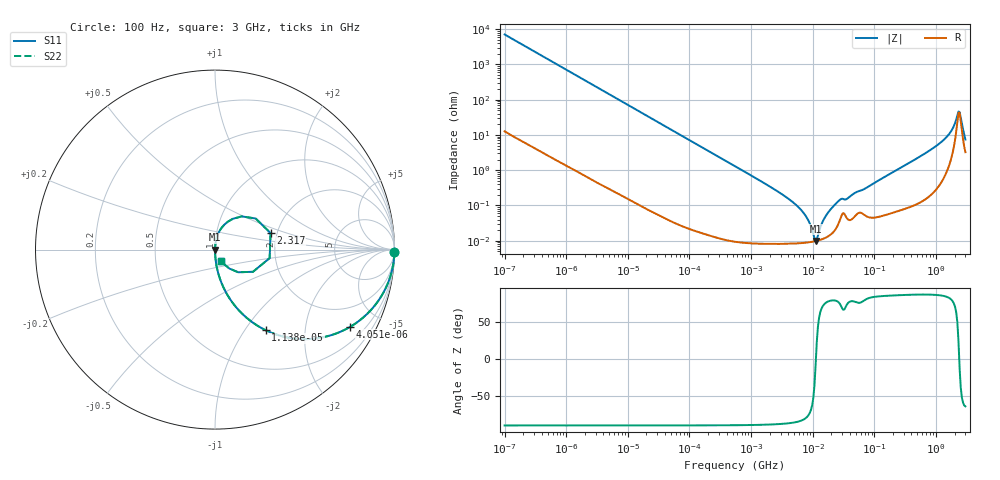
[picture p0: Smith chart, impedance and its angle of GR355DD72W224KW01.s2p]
!Murata Part Number: GR355DD72W224KW01
!These Parameters are Measured in Series Mode Connection
!Data Generated on Mar 13, 2026
!  o--ll--o
!Port1  Port2
!  o------o
!Operation Temp=25[degC], DC Bias Voltage=0[V]
!Freq. Start=100[Hz] Stop=3[GHz] 401[Steps]
# Hz S RI R 50
!Freq.(Hz) S11(Real) S11(Imag) S21(Real) S21(Imag) S12(Real) S12(Imag) S22(Real) S22(Imag)
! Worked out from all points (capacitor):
!   401 points, 100 Hz to 3 GHz, reference 50 ohm
!   read as one part in series: C = 225 nF near 109 Hz
!   lowest |Z| = 9.85 mohm at 11.14 MHz (marker M1)
!   series resonance near 11.26 MHz, so ESL is about 890 pH
!   S11 on the Smith chart (normalised r, x): 100 Hz: open; 4.051 kHz: 1.01, -3.51; 11.38 kHz: 1.00, -1.25; 2.317 GHz: 1.85, +0.38; 3 GHz: 1.06, -0.13
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100  0.9998 -0.0141  0.000225 0.0141  0.000225 0.0141  0.9998 -0.0141
536  0.9942 -0.0751  0.00581 0.0751  0.00581 0.0751  0.9942 -0.0751
1788  0.94 -0.2365  0.06 0.2365  0.06 0.2365  0.94 -0.2365
4051  0.7546 -0.4293  0.2454 0.4293  0.2454 0.4293  0.7546 -0.4293
11382  0.2818 -0.4488  0.7182 0.4488  0.7182 0.4488  0.2818 -0.4488
31977  0.0478 -0.2122  0.9522 0.2122  0.9522 0.2122  0.0478 -0.2122
102221  0.00507 -0.0695  0.9949 0.0695  0.9949 0.0695  0.00507 -0.0695
547723  0.000263 -0.013  0.9997 0.013  0.9997 0.013  0.000263 -0.013
4919190  8.45e-05 -0.00118  0.9999 0.00118  0.9999 0.00118  8.45e-05 -0.00118
7565221  8.79e-05 -0.000521  0.9999 0.000521  0.9999 0.000521  8.79e-05 -0.000521
9794414  9.34e-05 -0.000179  0.9999 0.000179  0.9999 0.000179  9.34e-05 -0.000179
1.11444e7  9.76e-05 -1.29e-05  0.9999 1.29e-05  0.9999 1.29e-05  9.76e-05 -1.29e-05
1.214626e7  0.000101 9.78e-05  0.9999 -9.78e-05  0.9999 -9.78e-05  0.000101 9.78e-05
1.641694e7  0.000123 0.000502  0.9999 -0.000502  0.9999 -0.000502  0.000123 0.000502
2.635803e7  0.000315 0.00131  0.9997 -0.00131  0.9997 -0.00131  0.000315 0.00131
1.751444e8  0.000637 0.00767  0.9994 -0.00767  0.9994 -0.00767  0.000637 0.00767
1.163803e9  0.00739 0.0583  0.9926 -0.0583  0.9926 -0.0583  0.00739 0.0583
1.789813e9  0.0388 0.124  0.9612 -0.124  0.9612 -0.124  0.0388 0.124
2.126076e9  0.1486 0.185  0.8514 -0.185  0.8514 -0.185  0.1486 0.185
2.317205e9  0.3097 0.0919  0.6903 -0.0919  0.6903 -0.0919  0.3097 0.0919
2.636591e9  0.1293 -0.1263  0.8707 0.1263  0.8707 0.1263  0.1293 -0.1263
3e9  0.0354 -0.0622  0.9646 0.0622  0.9646 0.0622  0.0354 -0.0622
